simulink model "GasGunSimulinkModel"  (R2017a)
settings: Solver=ode23t  StartTime=0.0  StopTime=1.5  RelTol=1e-3  EnableMultiTasking=on
undefined symbols (not defined in the file or in its folder): sigbuilder_block
libraries: Pneumatic_lib x9, fl_lib x6, nesl_utility x6, simulink x1

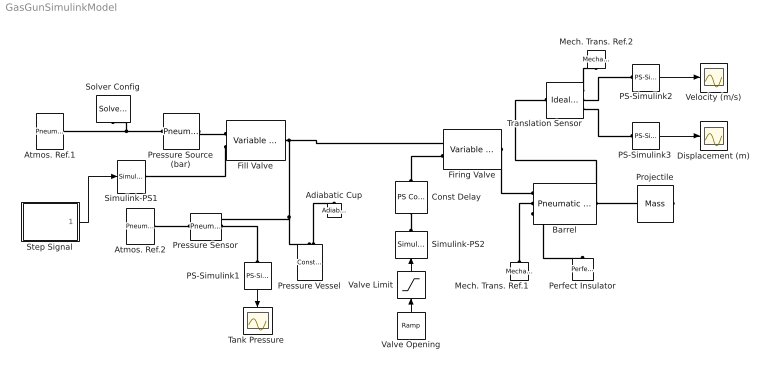
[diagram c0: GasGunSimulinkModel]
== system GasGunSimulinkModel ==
  Adiabatic Cup : Pneumatic_lib/Pneumatic Elements/Adiabatic Cup
  Atmos. Ref.1 : Pneumatic_lib/Pneumatic Elements/Pneumatic Atmospheric Reference
  Atmos. Ref.2 : Pneumatic_lib/Pneumatic Elements/Pneumatic Atmospheric Reference
  Barrel : Pneumatic_lib/Pneumatic Elements/Pneumatic Piston Chamber  Area=0.0019635 m^2  x0=0 m  V0=1e-05 m^3  or=1  pressure_specify=off  pressure_priority=High  pressure=1e+5 Pa  pressure_nominal_specify=off  pressure_nominal_unit=Pa  pressure_nominal_value=1  temperature_specify=off  temperature_priority=High  temperature=300 K  temperature_nominal_specify=off  temperature_nominal_unit=K  temperature_nominal_value=1  gas_flow_specify=off  gas_flow_priority=High  gas_flow=0 kg/s  gas_flow_nominal_specify=off  gas_flow_nominal_unit=kg/s  gas_flow_nominal_value=1  heat_flow_specify=off  heat_flow_priority=High  heat_flow=0 J/s  heat_flow_nominal_specify=off  heat_flow_nominal_unit=J/s  heat_flow_nominal_value=1  heat_exch_flow_specify=off  heat_exch_flow_priority=High  heat_exch_flow=0 J/s  heat_exch_flow_nominal_specify=off  heat_exch_flow_nominal_unit=J/s  heat_exch_flow_nominal_value=1  velocity_specify=off  velocity_priority=High  velocity=0 m/s  velocity_nominal_specify=off  velocity_nominal_unit=m/s  velocity_nominal_value=1  force_specify=off  force_priority=High  force=0 N  force_nominal_specify=off  force_nominal_unit=N  force_nominal_value=1
  Const Delay : fl_lib/Physical Signals/Delays/PS Constant Delay  InputHistory=0.0  DelayTime=0.5 s
  Displacement (m) : Scope
  Fill Valve : Pneumatic_lib/Pneumatic Elements/Variable Area Pneumatic Orifice  Cd=1  Area0=1e-13 m^2  G_specify=off  G_priority=High  G=0 kg/s  G_nominal_specify=off  G_nominal_unit=kg/s  G_nominal_value=1  Q1_specify=off  Q1_priority=High  Q1=0 J/s  Q1_nominal_specify=off  Q1_nominal_unit=J/s  Q1_nominal_value=1  Q2_specify=off  Q2_priority=High  Q2=0 J/s  Q2_nominal_specify=off  Q2_nominal_unit=J/s  Q2_nominal_value=1  p1_specify=off  p1_priority=High  p1=1e+5 Pa  p1_nominal_specify=off  p1_nominal_unit=Pa  p1_nominal_value=1  p2_specify=off  p2_priority=High  p2=1e+5 Pa  p2_nominal_specify=off  p2_nominal_unit=Pa  p2_nominal_value=1  T1_specify=off  T1_priority=High  T1=300 K  T1_nominal_specify=off  T1_nominal_unit=K  T1_nominal_value=1  T2_specify=off  T2_priority=High  T2=300 K  T2_nominal_specify=off  T2_nominal_unit=K  T2_nominal_value=1
  Firing Valve : Pneumatic_lib/Pneumatic Elements/Variable Area Pneumatic Orifice  Cd=0.64  Area0=1e-13 m^2  G_specify=off  G_priority=High  G=0 kg/s  G_nominal_specify=off  G_nominal_unit=kg/s  G_nominal_value=1  Q1_specify=off  Q1_priority=High  Q1=0 J/s  Q1_nominal_specify=off  Q1_nominal_unit=J/s  Q1_nominal_value=1  Q2_specify=off  Q2_priority=High  Q2=0 J/s  Q2_nominal_specify=off  Q2_nominal_unit=J/s  Q2_nominal_value=1  p1_specify=off  p1_priority=High  p1=1e+5 Pa  p1_nominal_specify=off  p1_nominal_unit=Pa  p1_nominal_value=1  p2_specify=off  p2_priority=High  p2=1e+5 Pa  p2_nominal_specify=off  p2_nominal_unit=Pa  p2_nominal_value=1  T1_specify=off  T1_priority=High  T1=300 K  T1_nominal_specify=off  T1_nominal_unit=K  T1_nominal_value=1  T2_specify=off  T2_priority=High  T2=300 K  T2_nominal_specify=off  T2_nominal_unit=K  T2_nominal_value=1
  Mech. Trans. Ref.1 : fl_lib/Mechanical/Translational Elements/Mechanical Translational Reference
  Mech. Trans. Ref.2 : fl_lib/Mechanical/Translational Elements/Mechanical Translational Reference
  PS-Simulink1 : nesl_utility/PS-Simulink Converter  PhysicalDomain=network_engine_domain  SubClassName=ps_output  LeftPortType=input  RightPortType=output  PseudoPeriodic=off  Frequencies=[]  Unit=1  AffineConversion=off
  PS-Simulink2 : nesl_utility/PS-Simulink Converter  PhysicalDomain=network_engine_domain  SubClassName=ps_output  LeftPortType=input  RightPortType=output  PseudoPeriodic=off  Frequencies=[]  Unit=1  AffineConversion=off
  "PS-Simulink3 " : nesl_utility/PS-Simulink Converter  PhysicalDomain=network_engine_domain  SubClassName=ps_output  LeftPortType=input  RightPortType=output  PseudoPeriodic=off  Frequencies=[]  Unit=1  AffineConversion=off
  Perfect Insulator : fl_lib/Thermal/Thermal Elements/Perfect Insulator  T_specify=off  T_priority=High  T=0 K  T_nominal_specify=off  T_nominal_unit=K  T_nominal_value=1
  Pressure Sensor : Pneumatic_lib/Pneumatic Sensors/Pneumatic Pressure & Temperature Sensor
  Pressure Source (bar) : Pneumatic_lib/Pneumatic Sources/Pneumatic Pressure Source  pressure_difference_reference=8 bar
  Pressure Vessel : Pneumatic_lib/Pneumatic Elements/Constant Volume Pneumatic Chamber  Volume=0.02 m^3  pressure_specify=off  pressure_priority=High  pressure=1e+5 Pa  pressure_nominal_specify=off  pressure_nominal_unit=Pa  pressure_nominal_value=1  temperature_specify=off  temperature_priority=High  temperature=300 K  temperature_nominal_specify=off  temperature_nominal_unit=K  temperature_nominal_value=1  gas_flow_specify=off  gas_flow_priority=High  gas_flow=0 kg/s  gas_flow_nominal_specify=off  gas_flow_nominal_unit=kg/s  gas_flow_nominal_value=1  heat_flow_specify=off  heat_flow_priority=High  heat_flow=0 J/s  heat_flow_nominal_specify=off  heat_flow_nominal_unit=J/s  heat_flow_nominal_value=1  heat_exch_flow_specify=off  heat_exch_flow_priority=High  heat_exch_flow=0 J/s  heat_exch_flow_nominal_specify=off  heat_exch_flow_nominal_unit=J/s  heat_exch_flow_nominal_value=1
  Projectile : fl_lib/Mechanical/Translational Elements/Mass  mass=0.38 kg  v_specify=off  v_priority=High  v=0 m/s  v_nominal_specify=off  v_nominal_unit=m/s  v_nominal_value=1  f_specify=off  f_priority=High  f=0 N  f_nominal_specify=off  f_nominal_unit=N  f_nominal_value=1
  Simulink-PS1 : nesl_utility/Simulink-PS Converter  PhysicalDomain=network_engine_domain  SubClassName=ps_input  LeftPortType=input  RightPortType=output  PseudoPeriodic=off  Frequencies=[]  NoiseDistribution=none  NoiseParameters=[]  Unit=1  AffineConversion=off  FilteringAndDerivatives=zero  SimscapeFilterOrder=1  InputFilterTimeConstant=0.001  UdotUserProvided=1
  "Simulink-PS2 " : nesl_utility/Simulink-PS Converter  PhysicalDomain=network_engine_domain  SubClassName=ps_input  LeftPortType=input  RightPortType=output  PseudoPeriodic=off  Frequencies=[]  NoiseDistribution=none  NoiseParameters=[]  Unit=1  AffineConversion=off  FilteringAndDerivatives=zero  SimscapeFilterOrder=1  InputFilterTimeConstant=0.001  UdotUserProvided=1
  Solver Config : nesl_utility/Solver Configuration  PhysicalDomain=network_engine_domain  SubClassName=solver  LeftPortType=input  RightPortType=generic  Accelerate=off  Tones=[]  Harmonics=[]  SimulateNoise=off  Profile=off  UseLocalSampling=off  EnableSwitchedLinearOptims=on  FrequencyDomain=off  UseCCode=off  RelTol=0.001  AbsTol=1e-06  MinStep=1e-09  ToWorkspace=off  RevertToSquareIcSolve=off  NumHomotopyIterations=100  PhasorMode=off  PhasorModeNumHarmonics=1  OverrideAbsTol=off  DoDC=off  ResidualTolerance=1e-09  UseLocalSolver=off  LocalSolverChoice=NE_BACKWARD_EULER_ADVANCER  LocalSolverSampleTime=0.001  DoFixedCost=off  MaxNonlinIter=3  MaxModeIter=2  LinearAlgebra=Sparse  DelaysMemoryBudget=1024  AutomaticFiltering=on  FilteringTimeConstant=0.001
  Step Signal : Subsystem  Tag=STV Subsys  LoadFcn=sigbuilder_block('load');  StartFcn=sigbuilder_block('start');  StopFcn=sigbuilder_block('stop');  ClipboardFcn=sigbuilder_block('clipboard');
  "Tank Pressure " : Scope
  Translation Sensor : fl_lib/Mechanical/Mechanical Sensors/Ideal Translational Motion Sensor  offset=0 m
  Valve Limit : Saturate  UpperLimit=0.0019635
  Valve Opening : simulink/Sources/Ramp  slope=0.0098175  start=0  X0=0
  Velocity (m/s) : Scope
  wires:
  "PS-Simulink3 "/1 -> Displacement (m)/1
  PS-Simulink2/1 -> Velocity (m/s)/1
  PS-Simulink1/1 -> "Tank Pressure "/1
  Step Signal/1(Signal 1) -> Simulink-PS1/1
  Valve Opening/1 -> Valve Limit/1
  Valve Limit/1 -> "Simulink-PS2 "/1
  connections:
  Barrel/LConn3 -- Perfect Insulator/LConn1
  Mech. Trans. Ref.1/LConn1 -- Barrel/LConn2
  Translation Sensor/RConn2 -- PS-Simulink2/LConn1
  Translation Sensor/RConn3 -- "PS-Simulink3 "/LConn1
  Translation Sensor/RConn1 -- Mech. Trans. Ref.2/LConn1
  Barrel/RConn1 -- Translation Sensor/LConn1 -- Projectile/LConn1
  Pressure Source (bar)/RConn1 -- Atmos. Ref.1/LConn1 -- Solver Config/RConn1
  Pressure Sensor/LConn1 -- Atmos. Ref.2/LConn1
  Pressure Vessel/LConn2 -- Adiabatic Cup/LConn1
  Pressure Source (bar)/LConn1 -- Fill Valve/LConn1
  Fill Valve/LConn2 -- Simulink-PS1/RConn1
  Const Delay/LConn1 -- "Simulink-PS2 "/RConn1
  Const Delay/RConn1 -- Firing Valve/LConn2
  Firing Valve/RConn1 -- Barrel/LConn1
  Fill Valve/RConn1 -- Pressure Vessel/LConn1 -- Pressure Sensor/RConn1 -- Firing Valve/LConn1
  PS-Simulink1/LConn1 -- Pressure Sensor/RConn2

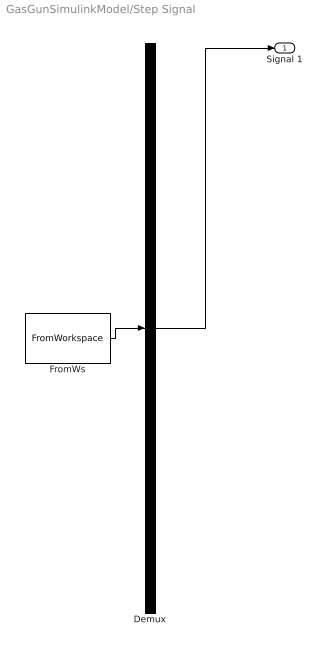
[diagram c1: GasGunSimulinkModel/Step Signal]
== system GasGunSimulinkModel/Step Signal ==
  Demux : Demux  Tag=STV Demux  Outputs=1
  FromWs : FromWorkspace  Tag=STV FromWs  VariableName=tuvar  SampleTime=0
  Signal 1 : Outport  Tag=STV Outport
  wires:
  Demux/1 -> Signal 1/1
  FromWs/1 -> Demux/1
